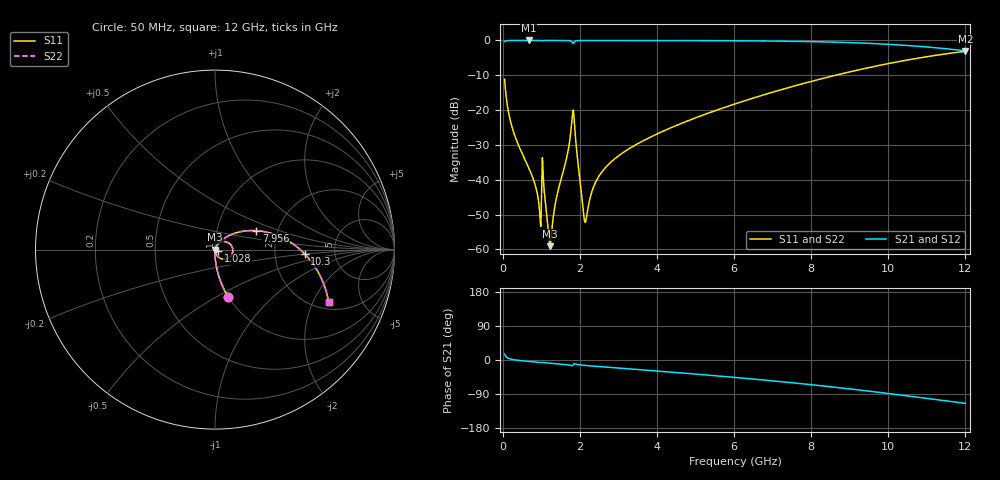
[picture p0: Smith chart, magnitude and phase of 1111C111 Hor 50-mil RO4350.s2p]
# GHz S MA R 50
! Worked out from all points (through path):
!   11951 points, 50 MHz to 12 GHz, reference 50 ohm
!   highest |S21| = -0.01 dB at 674 MHz (marker M1); lowest = -3.0 dB at 12 GHz (marker M2)
!   group delay of S21, straight-line fit = 26.3 ps
!   lowest |S11| = -59.1 dB at 1.226 GHz (marker M3), VSWR 1.00, Z = 50.1 - j0.0167 ohm
!   |S11| at or under -10 dB: start of sweep to 8.632 GHz
!   |S22| runs from -59.1 to -3.1 dB; largest |S21 - S12| = 0
!   S11 on the Smith chart (normalised r, x): 50 MHz: 1.00, -0.57; 1.028 GHz: 1.04, -0.02; 7.956 GHz: 1.55, +0.35; 10.3 GHz: 2.99, -0.20; 12 GHz: 2.32, -2.66
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0.05  0.2764 -74.2  0.9608 15.7  0.9608 15.7  0.2764 -74.2
0.253  0.0546 -88.1  0.998 1.4  0.998 1.4  0.0546 -88.1
0.674  0.01495 -90.8  0.9991 -3.7  0.9991 -3.7  0.01495 -90.8
0.85  0.008141 -89.0  0.999 -5.3  0.999 -5.3  0.008141 -89.0
0.946  0.004111 -79.6  0.9988 -6.1  0.9988 -6.1  0.004111 -79.6
1.028  0.02066 -23.7  0.9802 -6.6  0.9802 -6.6  0.02066 -23.7
1.072  0.007521 -81.7  0.9979 -6.8  0.9979 -6.8  0.007521 -81.7
1.176  0.002002 -63.9  0.9988 -7.8  0.9988 -7.8  0.002002 -63.9
1.226  0.001113 -8.6  0.9988 -8.3  0.9988 -8.3  0.001113 -8.6
1.813  0.09196 17.7  0.9213 -15.0  0.9213 -15.0  0.09196 17.7
1.866  0.05902 -57.5  0.959 -10.0  0.959 -10.0  0.05902 -57.5
2.042  0.006435 -70.6  0.9964 -13.4  0.9964 -13.4  0.006435 -70.6
2.152  0.002524 6.9  0.9975 -14.5  0.9975 -14.5  0.002524 6.9
2.36  0.007987 60.8  0.998 -16.2  0.998 -16.2  0.007987 60.8
2.645  0.01453 65.0  0.9981 -18.5  0.9981 -18.5  0.01453 65.0
4.034  0.04631 58.4  0.9968 -29.3  0.9968 -29.3  0.04631 58.4
6.025  0.1226 42.9  0.9896 -46.0  0.9896 -46.0  0.1226 42.9
7.956  0.2541 24.5  0.9633 -64.7  0.9633 -64.7  0.2541 24.5
8.017  0.2593 23.9  0.9618 -65.3  0.9618 -65.3  0.2593 23.9
10.009  0.4659 0.9  0.8794 -88.5  0.8794 -88.5  0.4659 0.9
10.305  0.5009 -2.8  0.8599 -92.2  0.8599 -92.2  0.5009 -2.8
12  0.6982 -24.9  0.7089 -114.4  0.7089 -114.4  0.6982 -24.9
